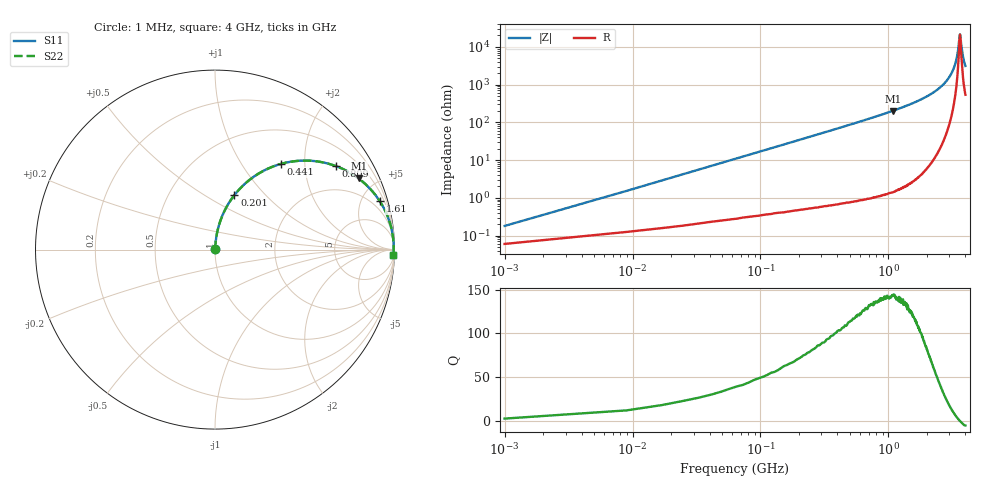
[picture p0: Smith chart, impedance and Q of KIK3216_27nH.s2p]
!version-2
!date-01.2022
!Series
# MHz S RI R 50
!Freq ReS11 ImS11 ReS21 ImS21 ReS12 ImS12 ReS22 ImS22
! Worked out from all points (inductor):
!   501 points, 1 MHz to 4 GHz, reference 50 ohm
!   read as one part in series: L = 27 nH near 17 MHz
!   highest Q = 143 at 1.08 GHz (marker M1), where L = 29.7 nH
!   self-resonance near 3.625 GHz
!   S11 on the Smith chart (normalised r, x): 1 MHz: 1.00, +0.00; 201 MHz: 1.01, +0.68; 441 MHz: 1.01, +1.52; 809 MHz: 1.02, +2.89; 1.61 GHz: 1.06, +6.79; 4 GHz: 12, -62
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1  0.000607 0.00169  0.9994 -0.00169  0.9994 -0.00169  0.000607 0.00169
25  0.00364 0.0422  0.9964 -0.0422  0.9964 -0.0422  0.00364 0.0422
49  0.0093 0.0822  0.9907 -0.0822  0.9907 -0.0822  0.0093 0.0822
105  0.034 0.1716  0.966 -0.1716  0.966 -0.1716  0.034 0.1716
201  0.1081 0.3036  0.8919 -0.3036  0.8919 -0.3036  0.1081 0.3036
441  0.3669 0.4773  0.6331 -0.4773  0.6331 -0.4773  0.3669 0.4773
673  0.5824 0.4893  0.4176 -0.4893  0.4176 -0.4893  0.5824 0.4893
809  0.6747 0.4648  0.3253 -0.4648  0.3253 -0.4648  0.6747 0.4648
1080  0.8003 0.3963  0.1997 -0.3963  0.1997 -0.3963  0.8003 0.3963
1340  0.8714 0.3311  0.1286 -0.3311  0.1286 -0.3311  0.8714 0.3311
1610  0.9183 0.2696  0.0817 -0.2696  0.0817 -0.2696  0.9183 0.2696
2010  0.958 0.1945  0.042 -0.1945  0.042 -0.1945  0.958 0.1945
2670  0.987 0.0993  0.0131 -0.0993  0.0131 -0.0993  0.987 0.0993
3060  0.9933 0.0555  0.0067 -0.0555  0.0067 -0.0555  0.9933 0.0555
3340  0.9952 0.0271  0.00483 -0.0271  0.00483 -0.0271  0.9952 0.0271
3460  0.9954 0.0158  0.00457 -0.0158  0.00457 -0.0158  0.9954 0.0158
3540  0.9955 0.00838  0.00455 -0.00838  0.00455 -0.00838  0.9955 0.00838
3590  0.9954 0.00333  0.0046 -0.00333  0.0046 -0.00333  0.9954 0.00333
3630  0.9953 -0.000234  0.00467 0.000234  0.00467 0.000234  0.9953 -0.000234
3660  0.9953 -0.00235  0.00473 0.00235  0.00473 0.00235  0.9953 -0.00235
3790  0.9948 -0.0141  0.00521 0.0141  0.00521 0.0141  0.9948 -0.0141
4000  0.9935 -0.0311  0.00646 0.0311  0.00646 0.0311  0.9935 -0.0311
